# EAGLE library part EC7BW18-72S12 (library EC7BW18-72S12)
Isolated DC/DC Converters 20W 8.5-160Vin 12Vout 1.33A Source: Datasheet
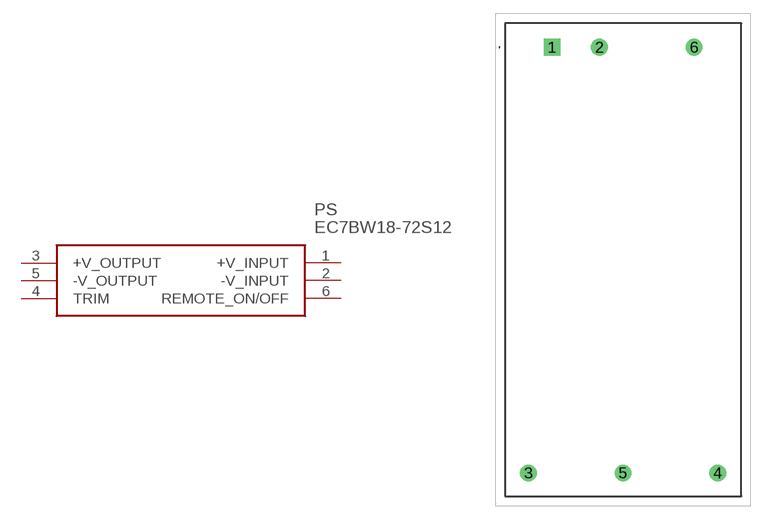
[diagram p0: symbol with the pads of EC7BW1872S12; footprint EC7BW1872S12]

Designator prefix PS

## EC7BW18-72S12 (Description: Isolated DC/DC Converters 20W 8.5-160Vin 12Vout 1.33A; Height: 10.7mm; Manufacturer_Name: Cincon; Manufacturer_Part_Number: EC7BW18-72S12; Mouser_Part_Number: 418-EC7BW18-72S12; Mouser_Price-Stock: https://www.mouser.co.uk/ProductDetail/Cincon/EC7BW18-72S12/?qs=wnTfsH77Xs4yy5rON%252BBkaQ%3D%3D)  [EC7BW1872S12]
1  +V_INPUT
2  -V_INPUT
3  +V_OUTPUT
4  TRIM
5  -V_OUTPUT
6  REMOTE_ON/OFF

## Footprint EC7BW1872S12 (pad centres in mm)
EC7BW18-72S12-1
drill 1.2 pad 1.8 square: 1 0,0
drill 1.2 pad 1.8: 2 5.08,0; 3 -2.54,-45.72; 4 17.78,-45.72; 5 7.62,-45.72; 6 15.24,0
